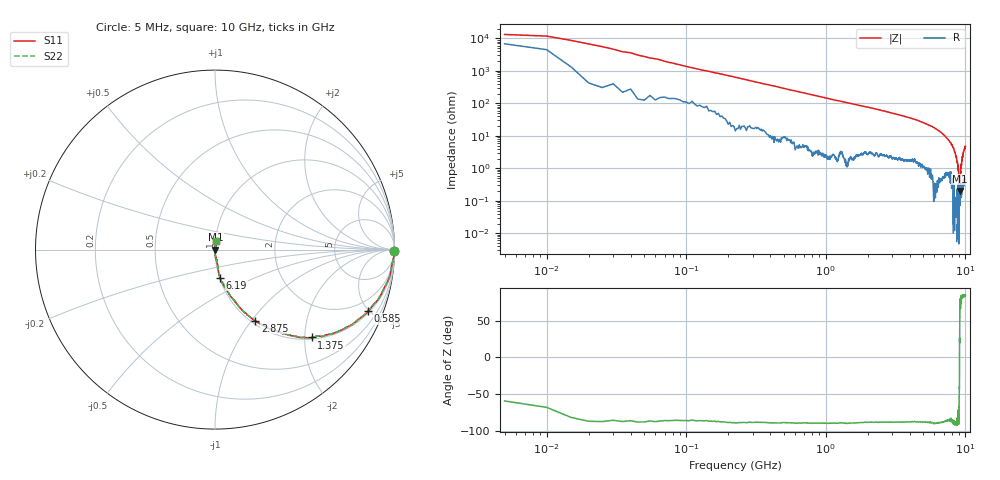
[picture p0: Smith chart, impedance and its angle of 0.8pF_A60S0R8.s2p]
! Amotech Co.,Ltd.
! http://www.amotech.co.kr/
! Part Number: A60S0R8
! These Parameters are Measured in Series Mode Connection
! Operation Temp=25[degC], DC Bias Voltage=0[V]
! Freq. Start=5[MHz] Stop=10[GHz], 2000[Steps]
! Date: Monday, July 13, 2020, 01:47:41
# GHZ S RI R 50.000000
!Freq.(Hz) S11(Real) S11(Imag) S21(Real) S21(Imag) S12(Real) S12(Imag) S22(Real) S22(Imag)
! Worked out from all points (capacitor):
!   2000 points, 5 MHz to 10 GHz, reference 50 ohm
!   read as one part in series: C = 1.16 pF near 55 MHz
!   lowest |Z| = 199 mohm at 9.085 GHz (marker M1)
!   series resonance near 9.078 GHz, so ESL is about 270 pH
!   S11 on the Smith chart (normalised r, x): 5 MHz: open; 585 MHz: 1.13, -4.96; 1.375 GHz: 1.04, -2.17; 2.875 GHz: 1.05, -1.05; 6.19 GHz: 1.00, -0.32; 10 GHz: 1.01, +0.10
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0.005  0.9961 -0.00642  0.00392 0.00642  0.00392 0.00642  0.9961 -0.00642
0.085  0.991 -0.0606  0.00898 0.0606  0.00898 0.0606  0.991 -0.0606
0.16  0.9802 -0.1105  0.0198 0.1105  0.0198 0.1105  0.9802 -0.1105
0.325  0.9427 -0.2126  0.0573 0.2126  0.0573 0.2126  0.9427 -0.2126
0.585  0.8541 -0.3406  0.1459 0.3406  0.1459 0.3406  0.8541 -0.3406
1.375  0.5392 -0.4895  0.4608 0.4895  0.4608 0.4895  0.5392 -0.4895
1.675  0.4496 -0.4838  0.5504 0.4838  0.5504 0.4838  0.4496 -0.4838
2.875  0.2252 -0.3956  0.7748 0.3956  0.7748 0.3956  0.2252 -0.3956
3.34  0.1759 -0.3576  0.8241 0.3576  0.8241 0.3576  0.1759 -0.3576
5.005  0.0694 -0.233  0.9306 0.233  0.9306 0.233  0.0694 -0.233
6.19  0.0275 -0.1565  0.9725 0.1565  0.9725 0.1565  0.0275 -0.1565
6.67  0.0207 -0.1256  0.9793 0.1256  0.9793 0.1256  0.0207 -0.1256
7.85  0.00903 -0.0602  0.991 0.0602  0.991 0.0602  0.00903 -0.0602
8.335  0.00103 -0.0339  0.999 0.0339  0.999 0.0339  0.00103 -0.0339
8.615  0.000883 -0.0223  0.9991 0.0223  0.9991 0.0223  0.000883 -0.0223
8.79  0.000253 -0.0136  0.9997 0.0136  0.9997 0.0136  0.000253 -0.0136
8.9  0.00236 -0.0084  0.9976 0.0084  0.9976 0.0084  0.00236 -0.0084
9.085  0.00192 0.000521  0.9981 -0.000521  0.9981 -0.000521  0.00192 0.000521
9.135  0.000808 0.00334  0.9992 -0.00334  0.9992 -0.00334  0.000808 0.00334
9.315  0.0025 0.0111  0.9975 -0.0111  0.9975 -0.0111  0.0025 0.0111
9.475  0.00262 0.0198  0.9974 -0.0198  0.9974 -0.0198  0.00262 0.0198
10  0.00657 0.0473  0.9934 -0.0473  0.9934 -0.0473  0.00657 0.0473
